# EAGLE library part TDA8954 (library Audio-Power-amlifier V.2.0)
The TDA8954 is a stereo or mono high-efficiency Class D audio power amplifier in a single IC featuring low power dissipation. It is designed to deliver up to 2 × 210 W into a 4 Ω load in a stereo Single-Ended (SE) application, or 1 × 420 W into an 8 Ω load in a mono Bridge-Tied Load (BTL) application.
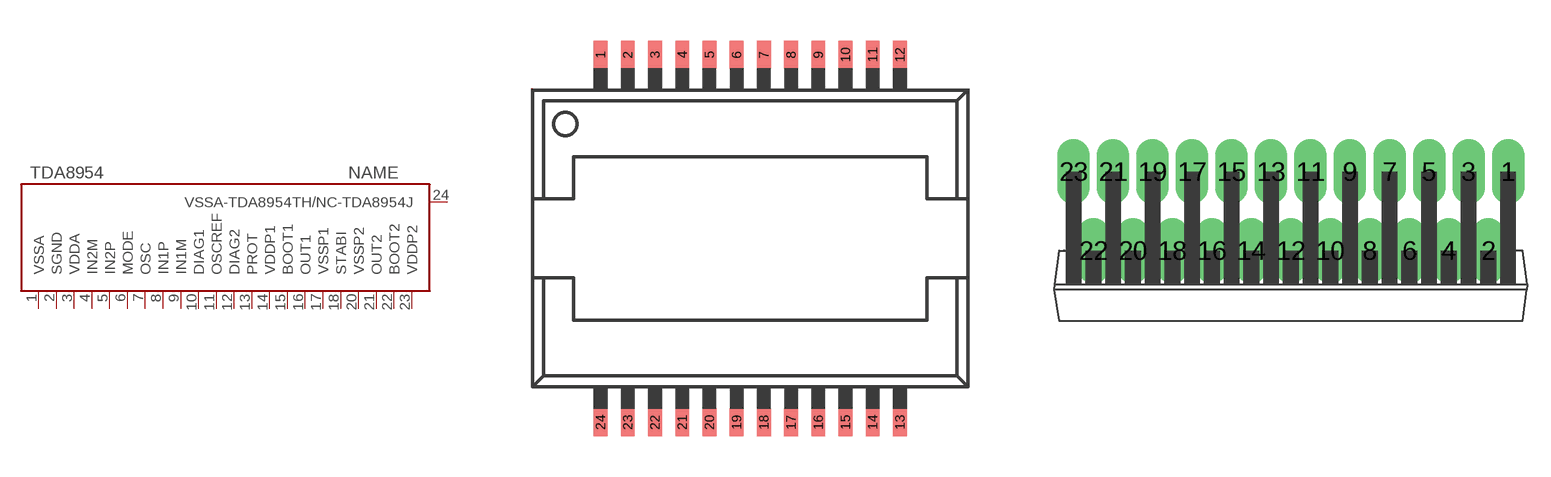
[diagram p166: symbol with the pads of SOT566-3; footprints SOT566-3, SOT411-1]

Designator prefix IC

## TDA8954TDA8954TH  [SOT566-3]
1  VSSA  pwr
2  SGND  pwr
3  VDDA  pwr
4  IN2M  in
5  IN2P  in
6  MODE  in
7  OSC  in
8  IN1P  in
9  IN1M  in
10  DIAG1  out
11  OSCREF
12  DIAG2  out
13  PROT
14  VDDP1  pwr
15  BOOT1
16  OUT1  out
17  VSSP1  pwr
18  STABI
20  VSSP2  pwr
21  OUT2  out
22  BOOT2
23  VDDP2  pwr
24  VSSA-TDA8954TH/NC-TDA8954J  pwr

## TDA8954TDA8954J  [SOT411-1]
1  MODE  in
2  IN2P  in
3  IN2M  in
4  VDDA  pwr
5  SGND  pwr
6  VSSA  pwr
7  VSSA-TDA8954TH/NC-TDA8954J  pwr
8  VDDP2  pwr
9  BOOT2
10  OUT2  out
11  VSSP2  pwr
12  STABI
13  VSSP1  pwr
14  OUT1  out
15  BOOT1
16  VDDP1  pwr
17  PROT
18  DIAG2  out
19  OSCREF
20  DIAG1  out
21  IN1M  in
22  IN1P  in
23  OSC  in

## Footprint SOT566-3 (pad centres in mm)
smd 0.508 x 1.016: 1 -5.5,6.75; 2 -4.5,6.75; 3 -3.5,6.75; 4 -2.5,6.75; 5 -1.5,6.75; 6 -0.5,6.75; 7 0.5,6.75; 8 1.5,6.75; 9 2.5,6.75; 10 3.5,6.75; 11 4.5,6.75; 12 5.5,6.75; 13 5.5,-6.75; 14 4.5,-6.75; 15 3.5,-6.75; 16 2.5,-6.75; 17 1.5,-6.75; 18 0.5,-6.75; 19 -0.5,-6.75; 20 -1.5,-6.75; 21 -2.5,-6.75; 22 -3.5,-6.75; 23 -4.5,-6.75; 24 -5.5,-6.75

## Footprint SOT411-1 (pad centres in mm)
drill 1.4 long: 1 13.97,5.08; 2 12.7,0; 3 11.43,5.08; 4 10.16,0; 5 8.89,5.08; 6 7.62,0; 7 6.35,5.08; 8 5.08,0; 9 3.81,5.08; 10 2.54,0; 11 1.27,5.08; 12 0,0; 13 -1.27,5.08; 14 -2.54,0; 15 -3.81,5.08; 16 -5.08,0; 17 -6.35,5.08; 18 -7.62,0; 19 -8.89,5.08; 20 -10.16,0; 21 -11.43,5.08; 22 -12.7,0; 23 -13.97,5.08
